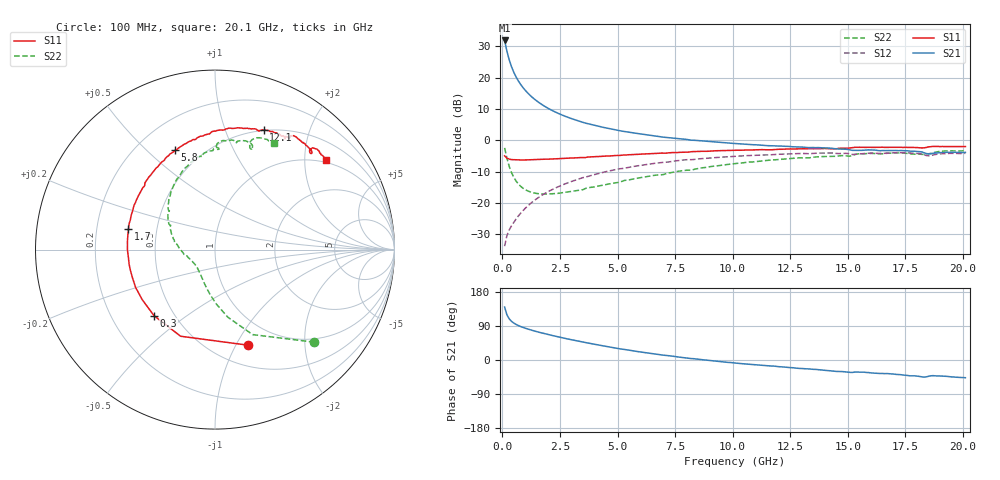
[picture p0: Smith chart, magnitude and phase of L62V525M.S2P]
!  Infineon Technologies AG
! BFR380L3 , PF131585-7, No.6, Th 09.10.01, soldered on pcb-board, measured with PP GSG850
!  Vce=2.5 V,  Ic=25.0 mA
! Common Emitter S-Parameters:  15. November 2001
#  GHz  S  MA  R  50
! f  S11  S21  S12  S22
! GHz  Mag  Ang  Mag  Ang  Mag  Ang  Mag  Ang
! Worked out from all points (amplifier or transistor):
!   201 points, 100 MHz to 20.1 GHz, reference 50 ohm
!   highest |S21| = 31.8 dB at 100 MHz (marker M1)
!   |S21| within 3 dB of that: start of sweep to 187.9 MHz
!   unconditionally stable (mu >= 1): 1.27 GHz to 4.389 GHz
!   at 3.4 GHz: K = 1.02, MAG = 8.3 dB, |S12| = -12.1 dB
!   at 10.1 GHz: K = 0.96, MSG = 2.0 dB, |S12| = -5.1 dB
!   at 20.1 GHz: K = 0.99, MSG = 0.1 dB, |S12| = -4.2 dB
!   S11 on the Smith chart (normalised r, x): 100 MHz: 0.72, -1.12; 300 MHz: 0.39, -0.38; 1.7 GHz: 0.34, +0.10; 5.8 GHz: 0.36, +0.61; 12.1 GHz: 0.50, +1.37; 20.1 GHz: 0.93, +2.53
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0.1  0.5642 -70.8  39.07 139.8  0.02048 61.5  0.7567 -43.0
0.2  0.5194 -111.7  26.37 119.2  0.03024 55.3  0.5178 -66.1
0.3  0.5009 -132.8  19.15 108.6  0.03722 55.3  0.3831 -79.3
0.4  0.4921 -145.6  14.87 102.0  0.04319 56.8  0.3047 -88.4
0.5  0.49 -154.4  12.11 97.4  0.04918 59.1  0.2563 -95.5
0.6  0.486 -160.9  10.18 93.8  0.0557 61.0  0.2235 -101.4
0.7  0.4853 -166.2  8.796 90.8  0.06224 62.2  0.2005 -106.6
0.8  0.4854 -170.4  7.742 88.2  0.06895 63.4  0.1839 -111.1
1  0.4859 -177.2  6.242 83.8  0.08263 64.7  0.1628 -119.1
1.2  0.4881 177.2  5.233 80.0  0.09646 65.1  0.1507 -125.8
1.4  0.491 172.7  4.512 76.5  0.1103 65.3  0.1437 -131.6
1.7  0.4956 166.6  3.746 71.6  0.1314 64.8  0.1394 -139.1
2.4  0.5076 154.3  2.714 61.4  0.1799 61.9  0.1421 -152.7
3.5  0.529 138.2  1.931 47.2  0.2538 55.3  0.163 -167.9
4.6  0.5608 124.7  1.545 34.9  0.3221 48.0  0.2001 177.3
5.8  0.5963 111.9  1.293 22.9  0.3876 39.8  0.2463 163.5
6.8  0.6205 102.3  1.148 14.1  0.4377 32.5  0.2812 152.1
10.1  0.6922 78.1  0.8876 -7.9  0.5547 11.0  0.4243 123.0
12.1  0.7186 67.8  0.808 -18.0  0.6004 -0.9  0.4977 106.9
13.5  0.7333 60.9  0.7655 -24.6  0.6185 -9.3  0.5353 97.1
16.8  0.7723 48.5  0.6856 -36.1  0.6252 -25.1  0.6232 76.8
20.1  0.7952 38.9  0.6415 -46.7  0.6199 -38.6  0.6798 61.1
